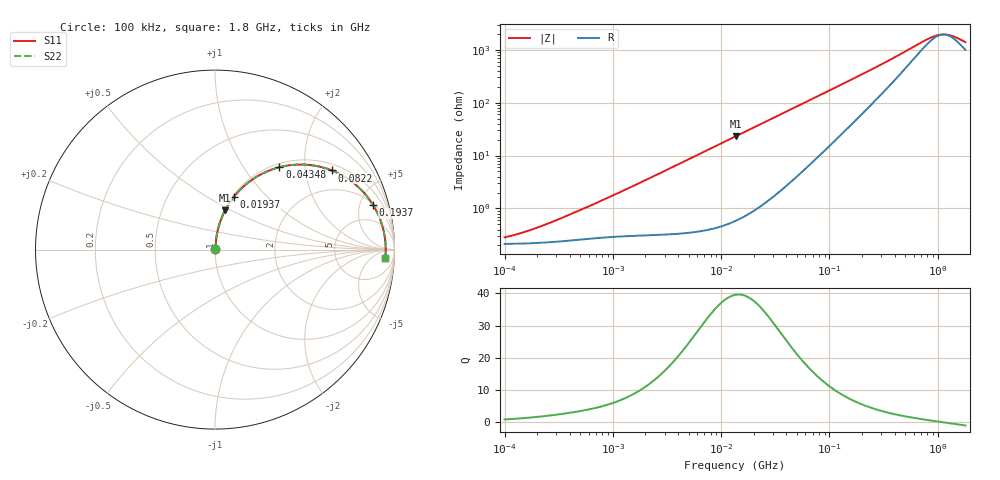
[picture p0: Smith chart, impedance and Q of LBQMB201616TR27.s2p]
! LBQMB201616TR27  S-PARAMETER MODEL  ( General Type )
! Model Generated by TAIYO YUDEN Corporation (http://www.ty-top.com)
! Version 1.0
! TAIYO YUDEN Control No. 191025NI43SB-FBB
! Copyright(c) 2019 TAIYO YUDEN CO.,LTD. All Rights Reserved.
! Product Description (link to TY-COMPAS)
! https://ds.yuden.co.jp/TYCOMPAS/or/detail?pn=LBQMB201616TR27J&u=M
! Products Name : Inductors
! Characteristics :
!  Inductance : 0.27 uH , SRF(min) : 425 MHz , DC Resistance(max) : 0.273 Ohm , Rated Current : 510 mA
!  Case Size : 2.0 x 1.6 / 0.079 x 0.063 [mm/inch] , Thickness : 1.6 / 0.063 [mm/inch]
!  (Conditions: Temperature = 25 degC , DC Bias Current/Voltage = 0A / 0V)
! External Node Assignments :
!  1  o---GGG---o  2
! GND o---------o GND
! Frequency Range : 0.1MHz  -  1800MHz  [ 402 STEP ]
# MHz S RI R 50
! Freq[MHz].  S11 Real  S11 Imag  S21 Real  S21 Imag  S12 Real  S12 Imag  S22 Real  S22 Imag
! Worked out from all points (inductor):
!   401 points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, 100 kHz to 1.8 GHz, reference 50 ohm
!   read as one part in series: L = 285 nH near 414 kHz
!   highest Q = 39.6 at 13.75 MHz (marker M1), where L = 270 nH
!   self-resonance near 1.131 GHz
!   S11 on the Smith chart (normalised r, x): 100 kHz: 1.00, +0.00; 19.37 MHz: 1.02, +0.66; 43.48 MHz: 1.06, +1.48; 82.2 MHz: 1.21, +2.79; 193.7 MHz: 2.15, +6.57; 1.8 GHz: 21, -19
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0.1  0.00213 0.00187  0.9979 -0.00187  0.9979 -0.00187  0.00213 0.00187
0.134171  0.00216 0.0025  0.9978 -0.0025  0.9978 -0.0025  0.00216 0.0025
0.193745  0.00223 0.00359  0.9978 -0.00359  0.9978 -0.00359  0.00223 0.00359
0.516129  0.00267 0.00921  0.9973 -0.00921  0.9973 -0.00921  0.00267 0.00921
2.66389  0.00519 0.045  0.9948 -0.045  0.9948 -0.045  0.00519 0.045
6.434145  0.0154 0.1071  0.9846 -0.1071  0.9846 -0.1071  0.0154 0.1071
13.41641  0.0542 0.2141  0.9458 -0.2141  0.9458 -0.2141  0.0542 0.2141
13.74911  0.0566 0.2188  0.9434 -0.2188  0.9434 -0.2188  0.0566 0.2188
19.37354  0.1037 0.292  0.8963 -0.292  0.8963 -0.292  0.1037 0.292
28.66948  0.1989 0.3838  0.8011 -0.3838  0.8011 -0.3838  0.1989 0.3838
43.47794  0.3584 0.459  0.6416 -0.459  0.6416 -0.459  0.3584 0.459
55.54574  0.4724 0.474  0.5276 -0.474  0.5276 -0.474  0.4724 0.474
69.24595  0.5761 0.4636  0.4239 -0.4636  0.4239 -0.4636  0.5761 0.4636
82.19808  0.6511 0.441  0.3489 -0.441  0.3489 -0.441  0.6511 0.441
124.6553  0.7941 0.3525  0.2059 -0.3525  0.2059 -0.3525  0.7941 0.3525
193.7305  0.8815 0.2475  0.1185 -0.2475  0.1185 -0.2475  0.8815 0.2475
357.3983  0.9326 0.1317  0.0674 -0.1317  0.0674 -0.1317  0.9326 0.1317
782.6622  0.9499 0.0355  0.0501 -0.0355  0.0501 -0.0355  0.9499 0.0355
999.899  0.9511 0.0117  0.0489 -0.0117  0.0489 -0.0117  0.9511 0.0117
1130.179  0.9512 9.92e-05  0.0488 -9.92e-05  0.0488 -9.92e-05  0.9512 9.92e-05
1277.433  0.9511 -0.0115  0.0489 0.0115  0.0489 0.0115  0.9511 -0.0115
1800  0.9491 -0.0453  0.0509 0.0453  0.0509 0.0453  0.9491 -0.0453
